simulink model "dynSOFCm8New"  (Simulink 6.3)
settings: Solver=ode15s  StartTime=0.0  StopTime=5000  FixedStep=0.001  MinStep=1e-12  RelTol=1e-3
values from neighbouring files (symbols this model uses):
  C = 300e-2    (= 3)    [dynSOFC_par.m]
  Cpc = 740    [dynSOFC_par.m]
  Cpt = 1217.7    [dynSOFC_par.m]
  D_a = 0.273*2*r3    (= 0.006006)    [dynSOFC_par.m]
  D_c = 2*(r2-r1)    (= 0.00532)    [dynSOFC_par.m]
  delta = 5.67e-8    (= 5.67e-08)    [dynSOFC_par.m]
  Ea = 1.1e5    (= 110000)    [dynSOFC_par.m]
  Ec = 1.2e5    (= 120000)    [dynSOFC_par.m]
  Ems1 = 0.4    [dynSOFC_par.m]
  Ems2 = 0.9    [dynSOFC_par.m]
  F = 96487    [dynSOFC_par.m]
  F21 = 0.69    [dynSOFC_par.m]
  K = 10    [dynSOFC_par.m]
  L = 1.5    [dynSOFC_par.m]
  La = 0.1e-3    (= 0.0001)    [dynSOFC_par.m]
  Lc = 2.21e-3    (= 0.00221)    [dynSOFC_par.m]
  Le = 0.04e-3    (= 4e-05)    [dynSOFC_par.m]
  R = 8.314/101325    (= 8.20528003948e-05)    [dynSOFC_par.m]
  r0 = 5e-3    (= 0.005)    [dynSOFC_par.m]
  r1 = 6e-3    (= 0.006)    [dynSOFC_par.m]
  r2 = 8.66e-3    (= 0.00866)    [dynSOFC_par.m]
  r3 = 11e-3    (= 0.011)    [dynSOFC_par.m]
  Ro = 1e-6    (= 1e-06)    [dynSOFC_par.m]
  Rouc = 4592    [dynSOFC_par.m]
  Rout = 3900    [dynSOFC_par.m]
  X = z(i)    [Simulate.m]    (also in dynSOFC_par.m = 0)
  x_ini = x_INI(i,:)    [Simulate.m]    (also in dynSOFC_par.m = [)
  XCH4 = 0.173    [dynSOFC_par.m]
  XCO = 0.057    [dynSOFC_par.m]
  XCO2 = 0.228    [dynSOFC_par.m]
  XH2 = 0.258    [dynSOFC_par.m]
  XH2O = 0.284    [dynSOFC_par.m]
  XO2 = 0.21    [dynSOFC_par.m]
libraries: simulink x23
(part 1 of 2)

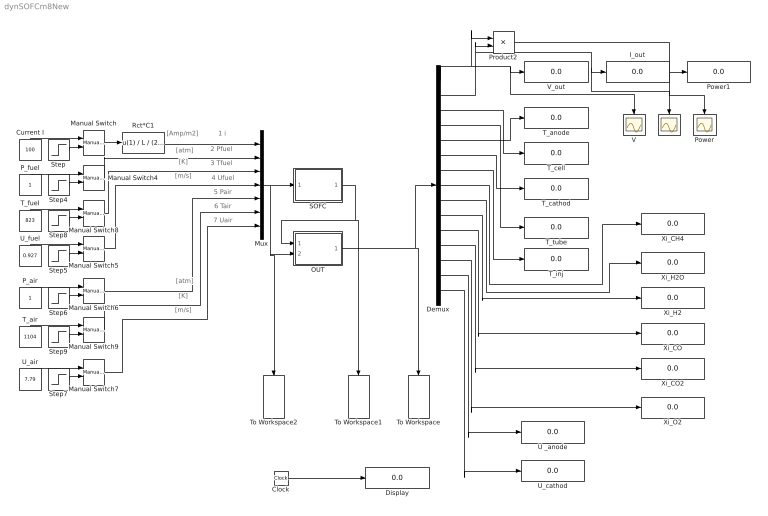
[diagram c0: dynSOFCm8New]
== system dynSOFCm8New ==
  note: [Amp/m2]
  note: [m/s]
  note: [atm]
  note: 1 i
  note: 3 Tfuel
  note: [K]
  note: 4 Ufuel
  note: 2 Pfuel
  note: 5 Pair
  note: 6 Tair
  note: 7 Uair
  note: [m/s]
  note: [K]
  note: [atm]
  Clock : Clock
  Current I : Constant  Orientation=up  Value=100
  Demux : Demux  Outputs=15
  Display : Display
  I : Scope
  I_out : Display
  Manual Switch{,4..6,8..9} (6 alike) : simulink/Signal Routing/Manual Switch  sw=1  action=0
  Manual Switch7 : simulink/Signal Routing/Manual Switch  sw=0  action=0
  Mux : Mux  Inputs=7
  OUT : Subsystem
  P_air : Constant  Orientation=up
  P_fuel : Constant  Orientation=up
  Power : Scope
  Power1 : Display
  Product2 : Product
  Rct*C1 : Fcn  Expr=u(1) / L / (2*pi*r3)
  SOFC : Subsystem
  Step : Step  Time=100  Before=100  After=200
  Step4 : Step  Time=100  Before=1  After=2
  Step5 : Step  Time=100  Before=0.97  After=2
  Step6 : Step  Time=100  Before=1  After=2
  Step7 : Step  Time=100  Before=7.79  After=23.37
  Step8 : Step  Time=100  Before=823  After=923
  Step9 : Step  Time=100  Before=1104  After=1204
  T_air : Constant  Orientation=up  Value=1104
  T_anode : Display
  T_cathod : Display
  T_cell : Display
  T_fuel : Constant  Orientation=up  Value=823
  T_inj : Display
  T_tube : Display
  To Workspace : ToWorkspace  VariableName=y  SampleTime=-1  SaveFormat=Array
  To Workspace1 : ToWorkspace  VariableName=x  SampleTime=-1  SaveFormat=Array
  To Workspace2 : ToWorkspace  VariableName=u  SaveFormat=Array
  U _anode : Display
  U_air : Constant  Orientation=up  Value=7.79
  U_cathod : Display
  U_fuel : Constant  Orientation=up  Value=0.927
  V : Scope
  V_out : Display
  Xi_CH4 : Display
  Xi_CO : Display
  Xi_CO2 : Display
  Xi_H2 : Display
  Xi_H2O : Display
  Xi_O2 : Display
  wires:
  Mux/1 -> SOFC/1(u), OUT/2(u), To Workspace2/1
  SOFC/1(x) -> OUT/1(x), To Workspace1/1
  OUT/1(y) -> Demux/1, To Workspace/1
  Demux/1 -> Product2/1, V_out/1, V/1
  Demux/2 -> Product2/2, I_out/1, I/1
  Current I/1 -> Manual Switch/1
  Step/1 -> Manual Switch/2
  Clock/1 -> Display/1
  P_fuel/1 -> Manual Switch4/1
  Step4/1 -> Manual Switch4/2
  U_fuel/1 -> Manual Switch5/1
  Step5/1 -> Manual Switch5/2
  P_air/1 -> Manual Switch6/1
  Step6/1 -> Manual Switch6/2
  U_air/1 -> Manual Switch7/1
  Step7/1 -> Manual Switch7/2
  T_fuel/1 -> Manual Switch8/1
  Step8/1 -> Manual Switch8/2
  T_air/1 -> Manual Switch9/1
  Step9/1 -> Manual Switch9/2
  Manual Switch5/1 -> Mux/4
  Manual Switch4/1 -> Mux/2
  Manual Switch8/1 -> Mux/3
  Manual Switch6/1 -> Mux/5
  Manual Switch9/1 -> Mux/6
  Manual Switch7/1 -> Mux/7
  Product2/1 -> Power1/1, Power/1
  Demux/3 -> T_cell/1
  Demux/4 -> T_tube/1
  Demux/5 -> T_anode/1
  Demux/6 -> T_cathod/1
  Demux/7 -> T_inj/1
  Demux/8 -> Xi_CH4/1
  Demux/9 -> Xi_H2O/1
  Demux/10 -> Xi_H2/1
  Demux/11 -> Xi_CO/1
  Demux/12 -> Xi_CO2/1
  Demux/13 -> Xi_O2/1
  Demux/14 -> U _anode/1
  Demux/15 -> U_cathod/1
  Manual Switch/1 -> Rct*C1/1
  Rct*C1/1 -> Mux/1

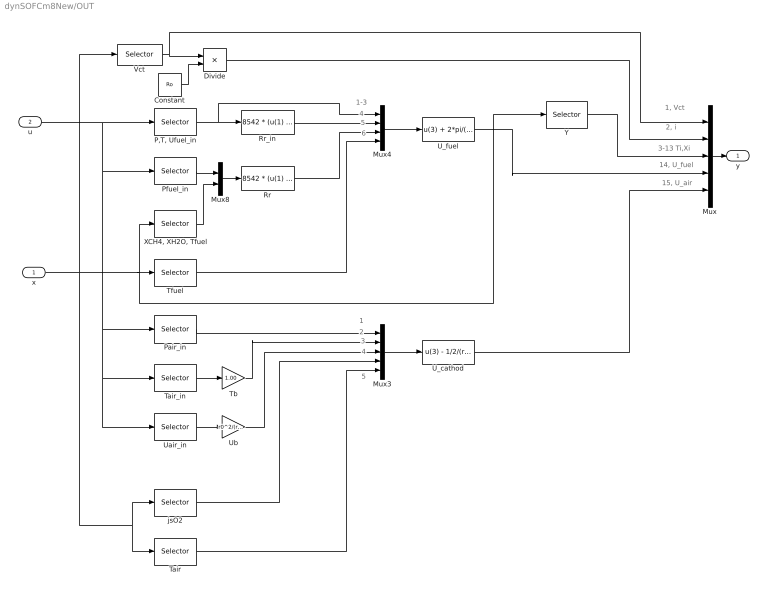
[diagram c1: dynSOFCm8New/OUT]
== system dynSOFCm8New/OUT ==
  note: 1-3
  note: 4
  note: 5
  note: 6
  note: 1
  note: 2
  note: 3
  note: 4
  note: 5
  note: 1, Vct
  note: 2, i
  note: 3-13 Ti,Xi
  note: 14, U_fuel
  note: 15, U_air
  x : Inport
  u : Inport  Port=2
  Constant : Constant  Value=Ro
  Divide : Product  Inputs=*/
  Mux : Mux  Inputs=5
  Mux3 : Mux  Inputs=5
  Mux4 : Mux
  Mux8 : Mux  Inputs=2
  "P,T, Ufuel_in" : Selector  Elements=[2 3 4]  InputPortWidth=7
  Pair_in : Selector  Elements=[5]  InputPortWidth=7
  Pfuel_in : Selector  Elements=[2]  InputPortWidth=7
  Rr : Fcn  Expr=8542 * (u(1) * u(2))^(0.85) * (u(1) * u(3))^(-0.35) * exp( -95e3 /(8.314*u(4)) )
  Rr_in : Fcn  Expr=8542 * (u(1) * XCH4)^(0.85) * (u(1) * XH2O)^(-0.35) * exp( -95e3 /(8.314*u(2)) )
  Tair : Selector  Elements=[18]  InputPortWidth=25
  Tair_in : Selector  Elements=[6]  InputPortWidth=7
  Tb : Gain  Gain=1.00
  Tfuel : Selector  Elements=[17]  InputPortWidth=25
  U_cathod : Fcn  Expr="u(3) - 1/2/(r2^2-r1^2)*(2*r1)  * R/u(1) * u(4) * ( u(2) + u(5)  ) * X"
  U_fuel : Fcn  Expr="u(3) + 2*pi/(4-pi)/r3  * R/u(1) * ( u(2) * u(4) + u(5) * u(6) ) * X"
  Uair_in : Selector  Elements=[7]  InputPortWidth=7
  Ub : Gain  Gain=r0^2/(r2^2-r1^2)
  Vct : Selector  Elements=[1]  InputPortWidth=25
  "XCH4, XH2O, Tfuel" : Selector  Elements=[20 21 17]  InputPortWidth=25
  Y : Selector  Elements=[15 16 17 18 19 20 21 22 23 24 25]  InputPortWidth=25
  jsO2 : Selector  Elements=[4]  InputPortWidth=25
  y : Outport
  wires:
  u/1 -> "P,T, Ufuel_in"/1, Pfuel_in/1, Pair_in/1, Uair_in/1, Tair_in/1
  Mux/1 -> y/1
  Tfuel/1 -> Mux4/4
  Pfuel_in/1 -> Mux8/1
  "XCH4, XH2O, Tfuel"/1 -> Mux8/2
  Mux8/1 -> Rr/1
  x/1 -> jsO2/1, Tair/1, Vct/1, "XCH4, XH2O, Tfuel"/1, Tfuel/1, Y/1
  "P,T, Ufuel_in"/1 -> Rr_in/1, Mux4/1
  Rr/1 -> Mux4/3
  Rr_in/1 -> Mux4/2
  Mux4/1 -> U_fuel/1
  Vct/1 -> Divide/1, Mux/1
  Constant/1 -> Divide/2
  jsO2/1 -> Mux3/4
  Pair_in/1 -> Mux3/1
  Mux3/1 -> U_cathod/1
  Uair_in/1 -> Ub/1
  Tair/1 -> Mux3/5
  Ub/1 -> Mux3/3
  Tair_in/1 -> Tb/1
  Tb/1 -> Mux3/2
  Divide/1 -> Mux/2
  Y/1 -> Mux/3
  U_fuel/1 -> Mux/4
  U_cathod/1 -> Mux/5

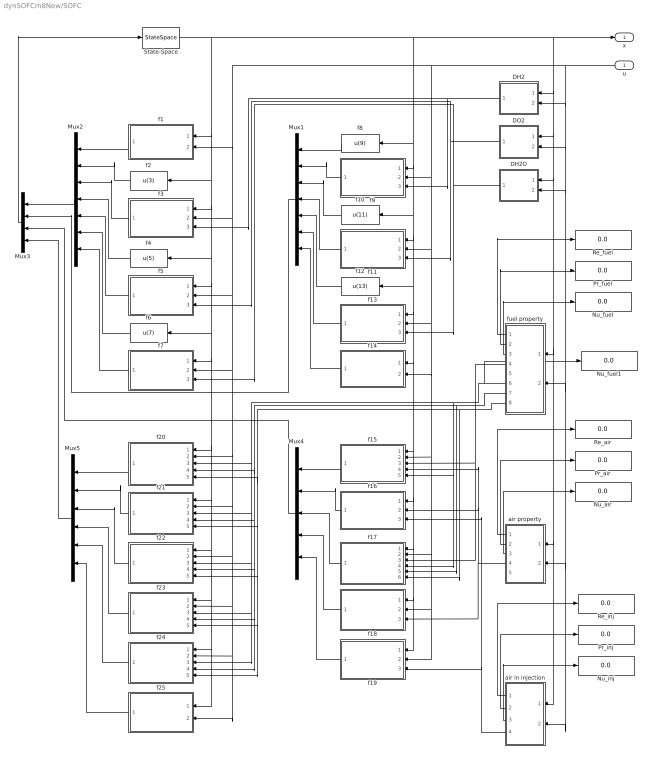
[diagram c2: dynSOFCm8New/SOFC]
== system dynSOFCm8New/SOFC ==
  u : Inport  Orientation=left
  DH2 : Subsystem  Orientation=left
  DH2O : Subsystem  Orientation=left
  DO2 : Subsystem  Orientation=left
  Mux1 : Mux  Orientation=left  Inputs=7
  Mux2 : Mux  Orientation=left  Inputs=7
  Mux3 : Mux  Orientation=left
  Mux4 : Mux  Orientation=left  Inputs=5
  Mux5 : Mux  Orientation=left  Inputs=6
  Nu_air : Display
  Nu_fuel : Display
  Nu_fuel1 : Display
  Nu_inj : Display
  Pr_air : Display
  Pr_fuel : Display
  Pr_inj : Display
  Re_air : Display
  Re_fuel : Display
  Re_inj : Display
  State-Space : StateSpace  A=zeros(25,25)  B=eye(25,25)  C=eye(25,25)  D=zeros(25,25)  X0=x_ini
  air in injection : Subsystem  Orientation=left
  air property : Subsystem  Orientation=left
  f1 : Subsystem  Orientation=left
  f10 : Fcn  Orientation=left  Expr=u(11)
  f11 : Subsystem  Orientation=left
  f12 : Fcn  Orientation=left  Expr=u(13)
  f13 : Subsystem  Orientation=left
  f14 : Subsystem  Orientation=left
  f15 : Subsystem  Orientation=left
  f16 : Subsystem  Orientation=left
  f17 : Subsystem  Orientation=left
  f18 : Subsystem  Orientation=left
  f19 : Subsystem  Orientation=left
  f2 : Fcn  Orientation=left  Expr=u(3)
  f20 : Subsystem  Orientation=left
  f21 : Subsystem  Orientation=left
  f22 : Subsystem  Orientation=left
  f23 : Subsystem  Orientation=left
  f24 : Subsystem  Orientation=left
  f25 : Subsystem  Orientation=left
  f3 : Subsystem  Orientation=left
  f4 : Fcn  Orientation=left  Expr=u(5)
  f5 : Subsystem  Orientation=left
  f6 : Fcn  Orientation=left  Expr=u(7)
  f7 : Subsystem  Orientation=left
  f8 : Fcn  Orientation=left  Expr=u(9)
  f9 : Subsystem  Orientation=left
  fuel property : Subsystem  Orientation=left
  x : Outport
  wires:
  State-Space/1 -> f1/1(x), f2/1, f3/1(x), f4/1, f6/1, f7/1(x), f21/1(x), f22/1(x), f23/1(x), f24/1(x), f25/1(x), f20/1(x), f5/1(x), f8/1, f9/1(x), f10/1, f11/1(x), f13/1(x), f14/1(x), f15/1(x), f16/1(x), f17/1(x), f18/1(x), f19/1(x), f12/1, x/1, DH2/1(x), DO2/1(x), DH2O/1(x), fuel property/1(x), air property/1(x), air in injection/1(x)
  f3/1(dot x3) -> Mux2/3
  f2/1 -> Mux2/2
  f1/1(dot x1) -> Mux2/1
  f4/1 -> Mux2/4
  f5/1(dot x5) -> Mux2/5
  f6/1 -> Mux2/6
  f7/1(dot x7) -> Mux2/7
  f8/1 -> Mux1/1
  f9/1(dot x9) -> Mux1/2
  f10/1 -> Mux1/3
  f11/1(dot x11) -> Mux1/4
  f12/1 -> Mux1/5
  f13/1(dot x13) -> Mux1/6
  f14/1(dot x14) -> Mux1/7
  Mux2/1 -> Mux3/1
  Mux3/1 -> State-Space/1
  u/1 -> f1/2(u), f3/2(u), f7/2(u), f21/2(u), f22/2(u), f23/2(u), f24/2(u), f25/2(u), f20/2(u), f5/2(u), f9/2(u), f13/2(u), f14/2(u), f15/2(u), f17/2(u), f18/2(u), f19/2(u), f11/2(u), DH2/2(u), DO2/2(u), DH2O/2(u), fuel property/2(u), air property/2(u), air in injection/2(u)
  DH2/1(DH2) -> f3/3(DH2), f9/3(DH2)
  DO2/1(DO2) -> f11/3(DO2), f5/3(DO2)
  DH2O/1(DH2O) -> f7/3(DH2O), f13/3(DH2O)
  Mux1/1 -> Mux3/2
  fuel property/4(h_fuel) -> f15/3(ha), f17/3(ha)
  air in injection/4(h_inj) -> f19/3(ht), f16/3(h_t)
  f15/1(dot x15) -> Mux4/1
  f16/1(dot x16) -> Mux4/2
  f17/1(dot x17) -> Mux4/3
  f18/1(dot x18) -> Mux4/4
  f19/1(dot x19) -> Mux4/5
  f20/1(dot x20) -> Mux5/1
  f21/1(dot x21) -> Mux5/2
  f22/1(dot x22) -> Mux5/3
  f23/1(dot x23) -> Mux5/4
  f24/1(dot x24) -> Mux5/5
  Mux4/1 -> Mux3/3
  Mux5/1 -> Mux3/4
  air property/1(Re_air) -> Re_air/1
  air property/2(Pr_air) -> Pr_air/1
  fuel property/1(Re_fuel) -> Re_fuel/1
  fuel property/2(Pr_fuel) -> Pr_fuel/1
  fuel property/3(Nu_fuel) -> Nu_fuel/1
  air in injection/1(Re_inj) -> Re_inj/1
  air in injection/2(Pr_inj) -> Pr_inj/1
  f25/1(dot x25) -> Mux5/6
  air property/4(h_air) -> f18/3(hc), f16/2(hc), f15/4(hc)
  fuel property/6(r_ref) -> Nu_fuel1/1, f15/5(r_ref), f17/4(r_ref), f21/3(r_ref), f22/3(r_ref), f23/3(r_ref), f24/3(r_ref), f20/3(r_ref)
  fuel property/7(r_sft) -> f17/5(r_sft), f21/4(r_sft), f22/4(r_sft), f23/4(r_sft), f24/4(r_sft), f20/4(r_sft)
  fuel property/8(r_ref_in) -> f17/6(r_ref_in), f21/5(r_ref_in), f22/5(r_ref_in), f23/5(r_ref_in), f24/5(r_ref_in), f20/5(r_ref_in)
  air in injection/3(Nu_inj) -> Nu_inj/1
  air property/3(Nu_air) -> Nu_air/1

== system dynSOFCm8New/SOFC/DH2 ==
  x : Inport
  u : Inport  Port=2
  D : Fcn  Expr=4.17e-5*u(1)^1.75/u(2)/101325
  Mux1 : Mux  Inputs=2
  Pfuel : Selector  Elements=[2]  InputPortWidth=7
  Tcell : Selector  Elements=[15]  InputPortWidth=25
  DH2 : Outport
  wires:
  Pfuel/1 -> Mux1/2
  u/1 -> Pfuel/1
  x/1 -> Tcell/1
  Tcell/1 -> Mux1/1
  Mux1/1 -> D/1
  D/1 -> DH2/1

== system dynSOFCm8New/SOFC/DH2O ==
  x : Inport
  u : Inport  Port=2
  D : Fcn  Expr=4.17e-5*u(1)^1.75/u(2)/101325
  Mux1 : Mux  Inputs=2
  Pfuel : Selector  Elements=[2]  InputPortWidth=7
  Tcell : Selector  Elements=[15]  InputPortWidth=25
  DH2O : Outport
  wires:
  D/1 -> DH2O/1
  Mux1/1 -> D/1
  Tcell/1 -> Mux1/1
  x/1 -> Tcell/1
  u/1 -> Pfuel/1
  Pfuel/1 -> Mux1/2

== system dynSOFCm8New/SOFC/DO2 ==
  x : Inport
  u : Inport  Port=2
  D : Fcn  Expr=9.82e-6*u(1)^1.75/u(2)/101325
  Mux1 : Mux  Inputs=2
  Pair : Selector  Elements=[5]  InputPortWidth=7
  Tcell : Selector  Elements=[15]  InputPortWidth=25
  DO2 : Outport
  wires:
  D/1 -> DO2/1
  Mux1/1 -> D/1
  Tcell/1 -> Mux1/1
  x/1 -> Tcell/1
  u/1 -> Pair/1
  Pair/1 -> Mux1/2

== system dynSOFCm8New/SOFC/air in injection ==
  note: u7
  note: u5
  note: x19
  x : Inport
  u : Inport  Port=2
  Density : Fcn  Expr=u(3) * u(2)/(R*u(1)) / 1000
  Mux2 : Mux  Inputs=3
  Mux3 : Mux  Inputs=3
  Mux4 : Mux
  Mux5 : Mux  Orientation=left  Inputs=2
  Mux6 : Mux  Inputs=2
  Nusselt number : Fcn  Expr=0.332*u(2)^(1/3)*u(1)^(1/2)
  P_inj : Selector  Elements=[5]  InputPortWidth=7
  Prandtl number : Fcn  Expr=u(3)/u(1)*u(2)/u(4)
  Renold number : Fcn  Expr=D_c*u(1)*u(2)/u(3)
  T_air : Selector  Elements=[19]  InputPortWidth=25
  U_air : Selector  Elements=[7]  InputPortWidth=7
  conductivity : Fcn  Expr=0.01329 + 5.539e-5*u(1)
  "heat capacity, Cp" : Fcn  Expr=2.779e4 + 4.936*u(1)
  heat transfer coefficient : Fcn  Expr=u(1)*u(2)/D_c
  mole mass : Constant  Value=29
  viscosity : Fcn  Expr=1.514e-5 + 2.793e-8*u(1)
  Re_inj : Outport
  Pr_inj : Outport  Port=2
  Nu_inj : Outport  Port=3
  h_inj : Outport  Port=4
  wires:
  u/1 -> P_inj/1, U_air/1
  Nusselt number/1 -> Nu_inj/1, Mux6/1
  Mux5/1 -> Nusselt number/1
  Prandtl number/1 -> Mux5/2, Pr_inj/1
  conductivity/1 -> Mux4/4, Mux6/2
  "heat capacity, Cp"/1 -> Mux4/3
  Mux4/1 -> Prandtl number/1
  viscosity/1 -> Mux4/2, Mux3/3
  mole mass/1 -> Mux4/1, Mux2/3
  P_inj/1 -> Mux2/2
  Renold number/1 -> Mux5/1, Re_inj/1
  Mux3/1 -> Renold number/1
  Density/1 -> Mux3/2
  Mux2/1 -> Density/1
  U_air/1 -> Mux3/1
  T_air/1 -> Mux2/1, "heat capacity, Cp"/1, conductivity/1, viscosity/1
  Mux6/1 -> heat transfer coefficient/1
  heat transfer coefficient/1 -> h_inj/1
  x/1 -> T_air/1

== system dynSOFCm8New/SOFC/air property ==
  note: u7
  note: x25,18
  note: u5
  x : Inport
  u : Inport  Port=2
  Density : Fcn  Expr="((1-u(1)) *28 + u(1)*32) * u(3)/(R*u(2))  /1000"
  Mole Mass : Fcn  Expr=(1 - u(1)) *28 + u(1)*32
  Mux1 : Mux  Inputs=2
  Mux3 : Mux  Inputs=3
  Mux4 : Mux
  Mux5 : Mux  Orientation=left  Inputs=2
  Mux6 : Mux  Inputs=2
  Nusselt number : Fcn  Expr=0.332*u(2)^(1/3)*u(1)^(1/2)
  P_air_in : Selector  Elements=[5]  InputPortWidth=7
  Prandtl number : Fcn  Expr=u(3)/u(1)*u(2)/u(4)
  Renold number : Fcn  Expr=D_c*u(1)*u(2)/u(3)
  U_air_in : Selector  Elements=[7]  InputPortWidth=7
  Ub : Gain  Gain=r0^2/(r2^2-r1^2)
  XO2,T_air : Selector  Elements=[25,18]  InputPortWidth=25
  conductivity : Fcn  Expr=0.01329 + 5.539e-5*u(2)
  "heat capacity, Cp" : Fcn  Expr=2.779e4 + 4.936*u(2)
  heat transfer coefficient : Fcn  Expr=u(1)*u(2)/D_c
  viscosity : Fcn  Expr=1.514e-5 + 2.793e-8*u(2)
  Re_air : Outport
  Pr_air : Outport  Port=2
  Nu_air : Outport  Port=3
  h_air : Outport  Port=4
  "Cp, air" : Outport  Port=5
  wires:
  heat transfer coefficient/1 -> h_air/1
  Mux6/1 -> heat transfer coefficient/1
  Density/1 -> Mux3/2
  Mux3/1 -> Renold number/1
  Renold number/1 -> Re_air/1, Mux5/1
  x/1 -> XO2,T_air/1
  Mole Mass/1 -> Mux4/1
  viscosity/1 -> Mux3/3, Mux4/2
  Mux4/1 -> Prandtl number/1
  "heat capacity, Cp"/1 -> Mux4/3, "Cp, air"/1
  conductivity/1 -> Mux6/2, Mux4/4
  Prandtl number/1 -> Pr_air/1, Mux5/2
  Mux5/1 -> Nusselt number/1
  Nusselt number/1 -> Mux6/1, Nu_air/1
  Mux1/1 -> Mole Mass/1, viscosity/1, "heat capacity, Cp"/1, conductivity/1, Density/1
  XO2,T_air/1 -> Mux1/1
  u/1 -> U_air_in/1, P_air_in/1
  P_air_in/1 -> Mux1/2
  U_air_in/1 -> Ub/1
  Ub/1 -> Mux3/1

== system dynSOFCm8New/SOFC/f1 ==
  note: E-Vct
  note: Tcell
  note: Vct
  note: i
  x : Inport
  u : Inport  Port=2
  Divide : Product  Inputs=*/
  E : Subsystem
  Gain1 : Gain  Gain=1/C
  I : Selector  Elements=[1]  InputPortWidth=7
  Rct*C : Fcn  Expr=2.94e-5*exp(10350/u(1)) *Le*C
  Sum : Sum  Inputs=|+-
  Sum1 : Sum  Inputs=|+-
  Tcell : Selector  Elements=[15]  InputPortWidth=25
  Vct : Selector  Elements=[1]  InputPortWidth=25
  dot x1 : Outport
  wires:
  E/1(E) -> Sum/1
  x/1 -> Vct/1, Tcell/1, E/1(x)
  Vct/1 -> Sum/2
  u/1 -> I/1, E/2(u)
  Gain1/1 -> Sum1/2
  Sum1/1 -> dot x1/1
  Sum/1 -> Divide/1
  Divide/1 -> Sum1/1
  Tcell/1 -> Rct*C/1
  Rct*C/1 -> Divide/2
  I/1 -> Gain1/1

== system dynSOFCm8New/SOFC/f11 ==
  note: 1-4
  note: 5
  note: 6
  note: 7-10
  note: x10,11,14,15
  note: u1
  note: x25
  note: u5
  note: pbO2
  note: dot ptO2
  note: ptO2
  note: i
  note: Vi
  note: Tcell
  x : Inport
  u : Inport  Port=2
  DO2 : Inport  Port=3
  Ex11 : Fcn  Expr="-u(7)*u(1) - u(8)*u(2)  + u(7)*u(5) - R*u(4)/(4*F)*( u(10)*u(6) + 4/Lc*(K*u(6)-u(3)) )"
  Mux : Mux
  Mux3 : Mux
  Mux4 : Mux  Inputs=2
  Pair_in : Selector  Elements=[5]  InputPortWidth=7
  XO2 : Selector  Elements=[25 ]  InputPortWidth=25
  a1 : Fcn  Expr=24*u(1)^2/(Lc^4)
  a2 : Fcn  Expr=12*u(1)/(Lc^2)
  a3 : Fcn  Expr=24*u(1)^2/(Lc^3)
  a4 : Fcn  Expr=24*u(1)/(Lc^3)
  i : Selector  Elements=[1]  InputPortWidth=7
  pbO2 : Fcn  Expr=u(2)*u(1)
  ptO2 : Selector  Elements=[10 11 14 15]  InputPortWidth=25
  dot x11 : Outport
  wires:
  DO2/1 -> a1/1, a2/1, a4/1, a3/1
  a1/1 -> Mux/1
  a2/1 -> Mux/2
  a3/1 -> Mux/3
  a4/1 -> Mux/4
  x/1 -> ptO2/1, XO2/1
  Mux3/1 -> Ex11/1
  Ex11/1 -> dot x11/1
  pbO2/1 -> Mux3/2
  u/1 -> Pair_in/1, i/1
  ptO2/1 -> Mux3/1
  XO2/1 -> Mux4/1
  Pair_in/1 -> Mux4/2
  Mux4/1 -> pbO2/1
  i/1 -> Mux3/3
  Mux/1 -> Mux3/4

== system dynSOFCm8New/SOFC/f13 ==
  note: 1-4
  note: 5
  note: 6
  note: 7-10
  note: x12,13,14,15
  note: u1
  note: x21
  note: u2
  note: pbH2O
  note: dot ptH2O
  note: ptH2O
  note: i
  note: Vi
  note: Tcell
  x : Inport
  u : Inport  Port=2
  DH2O : Inport  Port=3
  Ex9 : Fcn  Expr="-u(7)*u(1) - u(8)*u(2)  + u(7)*u(5) - R*u(4)/(2*F)*( u(10)*(-u(6)) - 4/La*(K*u(6)-u(3)) )"
  Mux : Mux
  Mux2 : Mux
  Mux4 : Mux  Inputs=2
  Pfuel_in : Selector  Elements=[2]  InputPortWidth=7
  XH2O : Selector  Elements=[21 ]  InputPortWidth=25
  a1 : Fcn  Expr=24*u(1)^2/(La^4)
  a2 : Fcn  Expr=12*u(1)/(La^2)
  a3 : Fcn  Expr=24*u(1)^2/(La^3)
  a4 : Fcn  Expr=24*u(1)/(La^3)
  i : Selector  Elements=[1]  InputPortWidth=7
  pbH2O : Fcn  Expr=u(2)*u(1)
  ptH2 : Selector  Elements=[12 13 14 15]  InputPortWidth=25
  dot x13 : Outport
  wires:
  DH2O/1 -> a1/1, a2/1, a4/1, a3/1
  a1/1 -> Mux/1
  a2/1 -> Mux/2
  a3/1 -> Mux/3
  a4/1 -> Mux/4
  x/1 -> ptH2/1, XH2O/1
  Mux2/1 -> Ex9/1
  Ex9/1 -> dot x13/1
  pbH2O/1 -> Mux2/2
  u/1 -> Pfuel_in/1, i/1
  ptH2/1 -> Mux2/1
  XH2O/1 -> Mux4/1
  Pfuel_in/1 -> Mux4/2
  Mux4/1 -> pbH2O/1
  i/1 -> Mux2/3
  Mux/1 -> Mux2/4

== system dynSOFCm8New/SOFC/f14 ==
  x : Inport
  u : Inport  Port=2
  Gain : Gain  Gain=K
  Gain1 : Gain  Gain=K^2
  Selector : Selector  Elements=[14]  InputPortWidth=25
  Selector1 : Selector  Elements=[1]  InputPortWidth=7
  Sum : Sum  Inputs=|-+
  dot x14 : Outport
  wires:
  Gain1/1 -> Sum/2
  Gain/1 -> Sum/1
  Selector1/1 -> Gain1/1
  Selector/1 -> Gain/1
  u/1 -> Selector1/1
  x/1 -> Selector/1
  Sum/1 -> dot x14/1

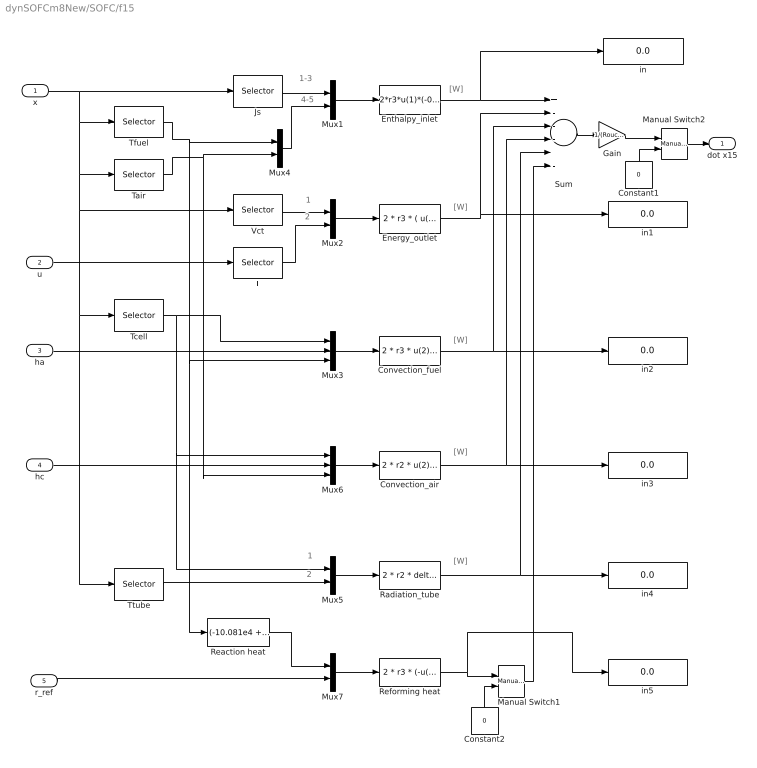
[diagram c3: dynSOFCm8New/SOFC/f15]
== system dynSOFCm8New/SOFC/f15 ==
  note: 1-3
  note: 4-5
  note: 1
  note: 2
  note: 1
  note: 2
  note: [W]
  note: [W]
  note: [W]
  note: [W]
  note: [W]
  x : Inport
  u : Inport  Port=2
  ha : Inport  Port=3
  hc : Inport  Port=4
  r_ref : Inport  Port=5
  Constant1 : Constant  Orientation=up  Value=0
  Constant2 : Constant  Orientation=up  Value=0
  Convection_air : Fcn  Expr=2 * r2 * u(2) * (u(1) - u(3))
  Convection_fuel : Fcn  Expr=2 * r3 * u(2) * (u(1) - u(3))
  Energy_outlet : Fcn  Expr=2 * r3 * ( u(1)*u(2) - u(2)^2 * Ro )
  Enthalpy_inlet : Fcn  Expr="2*r3*u(1)*(-0.9959e4+30.73*u(4)) + 2*r2*u(2)*(-1.2290e4+35.12*u(5))  + 2*r3*u(3)*(-25.790e4+42.47*u(4))"
  Gain : Gain  Gain=1/(Rouc*Cpc*(r3^2-r2^2))
  I : Selector  Elements=[1]  InputPortWidth=7
  Js : Selector  Elements=[2 4 6]  InputPortWidth=25
  Manual Switch1 : simulink/Signal Routing/Manual Switch  sw=1  action=0
  Manual Switch2 : simulink/Signal Routing/Manual Switch  sw=1  action=0
  Mux{1..2,4..5,7} (5 alike) : Mux  Inputs=2
  Mux3 : Mux  Inputs=3
  Mux6 : Mux  Inputs=3
  Radiation_tube : Fcn  Expr=2 * r2 * delta*(u(1)^4-u(2)^4)/((1-Ems2)/Ems2 + 1/F21 + (1-Ems1)/Ems1*(r2/r1)^2)
  Reaction heat : Fcn  Expr="(-10.081e4 + 62.12 * u(1)) +  (-25.79e4 + 42.47 * u(1)) - 3* (-0.9959e4 + 30.73*u(1))  -  (-12.150e4 + 31.81* u(1))"
  Reforming heat : Fcn  Expr=2 * r3 * (-u(1) * u(2))
  Sum : Sum  Inputs=+-----
  Tair : Selector  Elements=[18]  InputPortWidth=25
  Tcell : Selector  Elements=[15]  InputPortWidth=25
  Tfuel : Selector  Elements=[17]  InputPortWidth=25
  Ttube : Selector  Elements=[16]  InputPortWidth=25
  Vct : Selector  Elements=[1]  InputPortWidth=25
  in{,1..5} (6 alike) : Display
  dot x15 : Outport
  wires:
  x/1 -> Js/1, Tfuel/1, Vct/1, Tcell/1, Ttube/1, Tair/1
  Js/1 -> Mux1/1
  Mux1/1 -> Enthalpy_inlet/1
  Mux4/1 -> Mux1/2
  Vct/1 -> Mux2/1
  I/1 -> Mux2/2
  Mux2/1 -> Energy_outlet/1
  Mux3/1 -> Convection_fuel/1
  Mux5/1 -> Radiation_tube/1
  Tcell/1 -> Mux3/1, Mux5/1, Mux6/1
  u/1 -> I/1
  Enthalpy_inlet/1 -> Sum/1, in/1
  Energy_outlet/1 -> Sum/2, in1/1
  Convection_fuel/1 -> Sum/3, in2/1
  Convection_air/1 -> Sum/4, in3/1
  Radiation_tube/1 -> Sum/5, in4/1
  Mux6/1 -> Convection_air/1
  Tfuel/1 -> Mux4/1, Mux3/3, Reaction heat/1
  ha/1 -> Mux3/2
  hc/1 -> Mux6/2
  Tair/1 -> Mux6/3, Mux4/2
  Ttube/1 -> Mux5/2
  Mux7/1 -> Reforming heat/1
  r_ref/1 -> Mux7/2
  Reaction heat/1 -> Mux7/1
  Sum/1 -> Gain/1
  Gain/1 -> Manual Switch2/1
  Constant1/1 -> Manual Switch2/2
  Manual Switch2/1 -> dot x15/1
  Reforming heat/1 -> Manual Switch1/1, in5/1
  Constant2/1 -> Manual Switch1/2
  Manual Switch1/1 -> Sum/6

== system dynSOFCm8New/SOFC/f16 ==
  note: [W]
  note: [W]
  note: [W]
  x : Inport
  hc : Inport  Port=2
  h_t : Inport  Port=3
  Constant1 : Constant  Orientation=up  Value=0
  Convection_air : Fcn  Expr=2 * r1 * u(3) * (u(2) - u(1))
  Convection_inj : Fcn  Expr="2 * r0 *  u(3) * (u(1) - u(2))"
  Gain : Gain  Gain=1/(Rout*Cpt*(r1^2-r0^2))
  Manual Switch2 : simulink/Signal Routing/Manual Switch  sw=1  action=0
  Mux3 : Mux  Inputs=3
  Mux5 : Mux  Inputs=2
  Mux6 : Mux  Inputs=3
  Radiation_tube : Fcn  Expr=2 *r2 * delta*(u(1)^4-u(2)^4)/((1-Ems2)/Ems2 + 1/F21 + (1-Ems1)/Ems1*(r2/r1)^2)
  Sum : Sum  Inputs=+--
  Tair : Selector  Elements=[18]  InputPortWidth=25
  Tcell : Selector  Elements=[15]  InputPortWidth=25
  Tinj : Selector  Elements=[19]  InputPortWidth=25
  Ttube : Selector  Elements=[16]  InputPortWidth=25
  in1 : Display
  in2 : Display
  in3 : Display
  dot x16 : Outport
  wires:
  Mux6/1 -> Convection_inj/1
  Radiation_tube/1 -> in1/1, Sum/1
  Convection_inj/1 -> in3/1, Sum/3
  Convection_air/1 -> in2/1, Sum/2
  Mux5/1 -> Radiation_tube/1
  Mux3/1 -> Convection_air/1
  x/1 -> Tcell/1, Tair/1, Tinj/1, Ttube/1
  Tair/1 -> Mux3/1
  Tcell/1 -> Mux5/1
  Ttube/1 -> Mux5/2, Mux3/2, Mux6/1
  hc/1 -> Mux3/3
  Tinj/1 -> Mux6/2
  h_t/1 -> Mux6/3
  Sum/1 -> Gain/1
  Constant1/1 -> Manual Switch2/2
  Gain/1 -> Manual Switch2/1
  Manual Switch2/1 -> dot x16/1

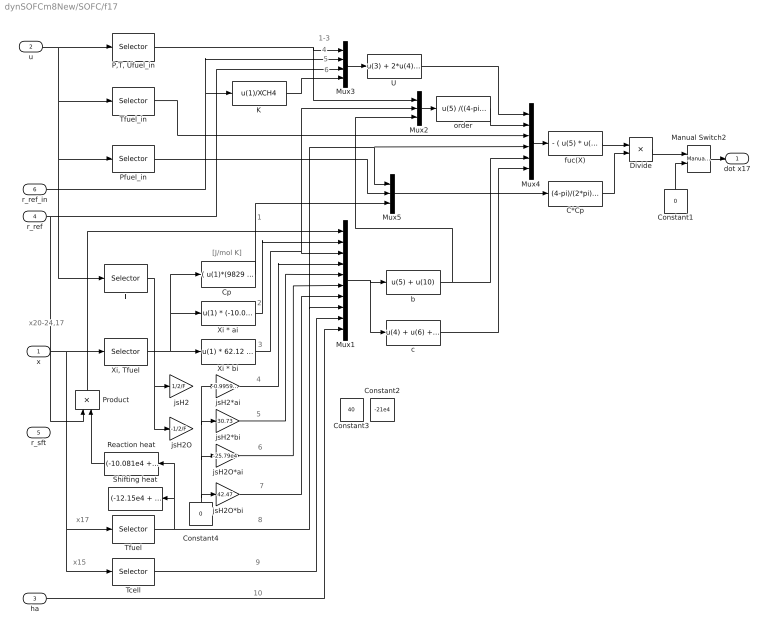
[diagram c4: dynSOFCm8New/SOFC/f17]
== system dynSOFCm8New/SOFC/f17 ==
  note: x20-24,17
  note: x17
  note: x15
  note: 1
  note: 2
  note: 3
  note: 4
  note: 5
  note: 6
  note: 7
  note: 8
  note: 9
  note: 10
  note: 1-3
  note: 4
  note: 5
  note: 6
  note: [J/mol K]
  x : Inport
  u : Inport  Port=2
  ha : Inport  Port=3
  r_ref : Inport  Port=4
  r_sft : Inport  Port=5
  r_ref_in : Inport  Port=6
  C*Cp : Fcn  Expr="(4-pi)/(2*pi)*r3 * u(2) / ( R * u(1) )  * u(3)"
  Constant1 : Constant  Orientation=up  Value=0
  Constant2 : Constant  Orientation=up  Value=-21e4
  Constant3 : Constant  Orientation=up  Value=40
  Constant4 : Constant  Orientation=up  Value=0
  "Cp " : Fcn  Expr="( u(1)*(9829 + 83.47*u(6) -0.02053*u(6)^2)  + u(2)*(2.906e4 + 12.15*u(6)) +  u(3)*(2.660e4 +3.719*u(6)) + u(4)*(2.797e4 + 5.019*u(6)) + u(5)*(3.200e4 + 31.01*u(6) - 0.008875*u(6)^2) )  / 1000"
  Divide : Product  Inputs=*/
  K : Fcn  Expr=u(1)/XCH4
  Manual Switch2 : simulink/Signal Routing/Manual Switch  sw=1  action=0
  Mux1 : Mux  Inputs=10
  Mux2 : Mux  Inputs=3
  Mux3 : Mux
  Mux4 : Mux  Inputs=6
  Mux5 : Mux  Inputs=3
  "P,T, Ufuel_in" : Selector  Elements=[2 3 4]  InputPortWidth=7
  Pfuel_in : Selector  Elements=[2]  InputPortWidth=7
  Product : Product  Orientation=up
  Reaction heat : Fcn  Orientation=left  Expr="(-10.081e4 + 62.12 * u(1)) +  (-25.79e4 + 42.47 * u(1)) - 3* (-0.9959e4 + 30.73*u(1))  -  (-12.150e4 + 31.81* u(1))"
  Shifting heat : Fcn  Orientation=left  Expr="(-12.15e4 + 31.81 * u(1)) +  (-25.79e4 + 42.47 * u(1)) - (-0.9959e4 + 30.73*u(1))  -  (-41.700e4 + 50.89* u(1))"
  Tcell : Selector  Elements=[15]  InputPortWidth=25
  Tfuel : Selector  Elements=[17]  InputPortWidth=25
  Tfuel_in : Selector  Elements=[3]  InputPortWidth=7
  U : Fcn  Expr=u(3) + 2*u(4)*u(3)/u(6) * ( 1- exp( -X/((4-pi)/(2*pi)*r3 * u(1) /R/u(2) * u(3) / u(6)) ) )
  Xi * ai : Fcn  Expr="u(1) * (-10.081e4)  + u(2) * (-25.79e4 ) + u(3) * (-0.9959e4) + u(4) * (-12.150e4) + u(5) * (-41.700e4 )"
  Xi * bi : Fcn  Expr="u(1) * 62.12 + u(2) * 42.47  + u(3) * 30.73 + u(4) * 31.81 + u(5) * 50.89"
  "Xi, Tfuel" : Selector  Elements=[20 21 22 23 24 17]  InputPortWidth=25
  b : Fcn  Expr=u(5) + u(10)
  c : Fcn  Expr=u(4) + u(6) + ( u(7) - u(10) ) * u(9) - u(1)*0
  fuc(X) : Fcn  Expr=- ( u(5) * u(4) +u(6) ) + ( u(5) * u(3) +u(6) ) * exp( - u(2)*X/u(1) )
  i : Selector  Elements=[1]  InputPortWidth=7
  jsH2 : Gain  Gain=1/2/F
  jsH2*ai : Gain  Gain=-0.9959e4
  jsH2*bi : Gain  Gain=30.73
  jsH2O : Gain  Gain=-1/2/F
  jsH2O*ai : Gain  Gain=-25.79e4
  jsH2O*bi : Gain  Gain=42.47
  order : Fcn  Expr=u(5) /((4-pi)/(2*pi)*r3 * u(1) /R/u(2) * u(4))
  dot x17 : Outport
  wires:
  Tcell/1 -> Mux1/9
  "Xi, Tfuel"/1 -> Xi * bi/1, "Cp "/1, Xi * ai/1
  Tfuel/1 -> Mux1/8, Mux4/4, Mux5/1, Shifting heat/1, Reaction heat/1
  ha/1 -> Mux1/10
  Pfuel_in/1 -> Mux5/2
  jsH2O*bi/1 -> Mux1/7
  x/1 -> "Xi, Tfuel"/1, Tfuel/1, Tcell/1
  "P,T, Ufuel_in"/1 -> Mux3/1, Mux2/1
  u/1 -> "P,T, Ufuel_in"/1, Tfuel_in/1, Pfuel_in/1, i/1
  jsH2*ai/1 -> Mux1/4
  jsH2*bi/1 -> Mux1/5
  jsH2O*ai/1 -> Mux1/6
  Mux1/1 -> b/1, c/1
  Mux3/1 -> U/1
  Mux2/1 -> order/1
  b/1 -> Mux4/5, Mux2/3
  Mux4/1 -> fuc(X)/1
  U/1 -> Mux4/1
  order/1 -> Mux4/2
  Tfuel_in/1 -> Mux4/3
  c/1 -> Mux4/6
  Mux5/1 -> C*Cp/1
  fuc(X)/1 -> Divide/1
  C*Cp/1 -> Divide/2
  "Cp "/1 -> Mux5/3
  Divide/1 -> Manual Switch2/1
  Constant1/1 -> Manual Switch2/2
  Manual Switch2/1 -> dot x17/1
  i/1 -> jsH2/1, jsH2O/1
  r_ref/1 -> Mux3/3, Product/1
  r_ref_in/1 -> Mux3/2, K/1
  Product/1 -> Mux1/1
  K/1 -> Mux3/4
  Reaction heat/1 -> Product/2
  Constant4/1 -> jsH2O*bi/1, jsH2O*ai/1, jsH2*bi/1, jsH2*ai/1
  Xi * ai/1 -> Mux1/2
  Xi * bi/1 -> Mux1/3, Mux2/2

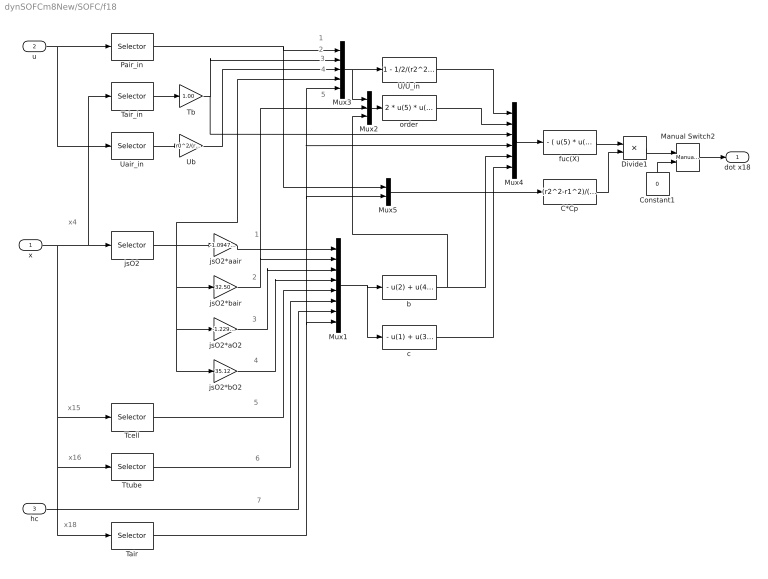
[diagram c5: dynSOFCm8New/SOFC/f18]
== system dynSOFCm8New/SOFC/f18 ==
  note: x4
  note: x15
  note: x16
  note: 1
  note: 4
  note: 5
  note: 6
  note: 7
  note: 1
  note: 2
  note: 3
  note: 4
  note: 2
  note: 3
  note: x18
  note: 5
  x : Inport
  u : Inport  Port=2
  hc : Inport  Port=3
  C*Cp : Fcn  Expr="(r2^2-r1^2)/(2*r1) * u(1) / ( R * u(2) )  * ( 2.7794e4 + 4.936 * u(2)) / 1000"
  Constant1 : Constant  Orientation=up  Value=0
  Divide1 : Product  Inputs=*/
  Manual Switch2 : simulink/Signal Routing/Manual Switch  sw=1  action=0
  Mux1 : Mux  Inputs=8
  Mux2 : Mux  Inputs=3
  Mux3 : Mux  Inputs=5
  Mux4 : Mux  Inputs=6
  Mux5 : Mux  Inputs=2
  Pair_in : Selector  Elements=[5]  InputPortWidth=7
  Tair : Selector  Elements=[18]  InputPortWidth=25
  Tair_in : Selector  Elements=[16]  InputPortWidth=25
  Tb : Gain  Gain=1.00
  Tcell : Selector  Elements=[15]  InputPortWidth=25
  Ttube : Selector  Elements=[16]  InputPortWidth=25
  U/U_in : Fcn  Expr="1 - 1/2/(r2^2-r1^2)*(2*r1)  * R/u(1)/u(3) * u(4) * ( u(2) + u(5)  ) * X"
  Uair_in : Selector  Elements=[7]  InputPortWidth=7
  Ub : Gain  Gain=r0^2/(r2^2-r1^2)
  b : Fcn  Expr=- u(2) + u(4) + u(7) + r2/r1*u(7)
  c : Fcn  Expr=- u(1) + u(3) - u(7)*u(5) - r2/r1*u(7)*u(6)
  fuc(X) : Fcn  Expr=- ( u(5) * u(4) +u(6) ) + ( u(5) * u(3) +u(6) ) * ( u(1) ^ u(2))
  jsO2 : Selector  Elements=[4]  InputPortWidth=25
  jsO2*aO2 : Gain  Gain=-1.229e4
  jsO2*aair : Gain  Gain=-1.0947e4
  jsO2*bO2 : Gain  Gain=35.12
  jsO2*bair : Gain  Gain=32.50
  order : Fcn  Expr="2 * u(5) * u(7) / ( u(6) * ( u(2)  + u(5) ) )"
  dot x18 : Outport
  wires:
  Ttube/1 -> Mux1/6
  Tcell/1 -> Mux1/5
  hc/1 -> Mux1/7
  jsO2/1 -> jsO2*aair/1, jsO2*bair/1, jsO2*aO2/1, jsO2*bO2/1, Mux3/4
  jsO2*bO2/1 -> Mux1/4
  x/1 -> Tcell/1, Ttube/1, Tair/1, jsO2/1, Tair_in/1
  Pair_in/1 -> Mux3/1, Mux5/1
  u/1 -> Pair_in/1, Uair_in/1
  jsO2*aair/1 -> Mux1/1
  jsO2*bair/1 -> Mux1/2, Mux2/2
  jsO2*aO2/1 -> Mux1/3
  Mux1/1 -> b/1, c/1
  Mux3/1 -> U/U_in/1, Mux2/1
  Mux2/1 -> order/1
  b/1 -> Mux2/3, Mux4/5
  Mux4/1 -> fuc(X)/1
  U/U_in/1 -> Mux4/1
  order/1 -> Mux4/2
  c/1 -> Mux4/6
  Mux5/1 -> C*Cp/1
  fuc(X)/1 -> Divide1/1
  C*Cp/1 -> Divide1/2
  Uair_in/1 -> Ub/1
  Tair/1 -> Mux1/8, Mux3/5, Mux4/4, Mux5/2
  Ub/1 -> Mux3/3
  Tair_in/1 -> Tb/1
  Tb/1 -> Mux3/2, Mux4/3
  Divide1/1 -> Manual Switch2/1
  Constant1/1 -> Manual Switch2/2
  Manual Switch2/1 -> dot x18/1

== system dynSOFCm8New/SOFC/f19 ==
  note: x19
  note: x16
  note: u5
  note: u6
  note: u7
  x : Inport
  u : Inport  Port=2
  ht : Inport  Port=3
  C*Cp : Fcn  Expr=r0/2 * u(1) / R / u(2) * ( 2.7794e4 + 4.936 * u(4)) / 1000
  Constant1 : Constant  Orientation=up  Value=0
  Divide : Product  Inputs=*/
  Manual Switch2 : simulink/Signal Routing/Manual Switch  sw=1  action=0
  Mux1 : Mux  Inputs=5
  Mux2 : Mux  Inputs=5
  Pair_in : Selector  Elements=[5]  InputPortWidth=7
  Tair_in : Selector  Elements=[6]  InputPortWidth=7
  Tinj : Selector  Elements=[19]  InputPortWidth=25
  Ttube : Selector  Elements=[16]  InputPortWidth=25
  Uair_in : Selector  Elements=[7]  InputPortWidth=7
  func : Fcn  Expr=u(4) * ( -u(2) + u(3) ) + u(4) * ( u(1) -u(3) ) * exp (u(5))
  in1 : Display
  order : Fcn  Expr=- 2/r0 * u(5) * R * u(4) / ( 32.5 * u(1) * u(3)) * (L-X)
  dot x19 : Outport
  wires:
  func/1 -> Divide/1
  u/1 -> Pair_in/1, Uair_in/1, Tair_in/1
  x/1 -> Tinj/1, Ttube/1
  Tinj/1 -> Mux1/4, Mux2/2
  ht/1 -> Mux1/5, Mux2/4
  Mux1/1 -> order/1, C*Cp/1
  Pair_in/1 -> Mux1/1
  Tair_in/1 -> Mux1/2, Mux2/1
  Uair_in/1 -> Mux1/3
  order/1 -> Mux2/5, in1/1
  Mux2/1 -> func/1
  Ttube/1 -> Mux2/3
  C*Cp/1 -> Divide/2
  Constant1/1 -> Manual Switch2/2
  Divide/1 -> Manual Switch2/1
  Manual Switch2/1 -> dot x19/1

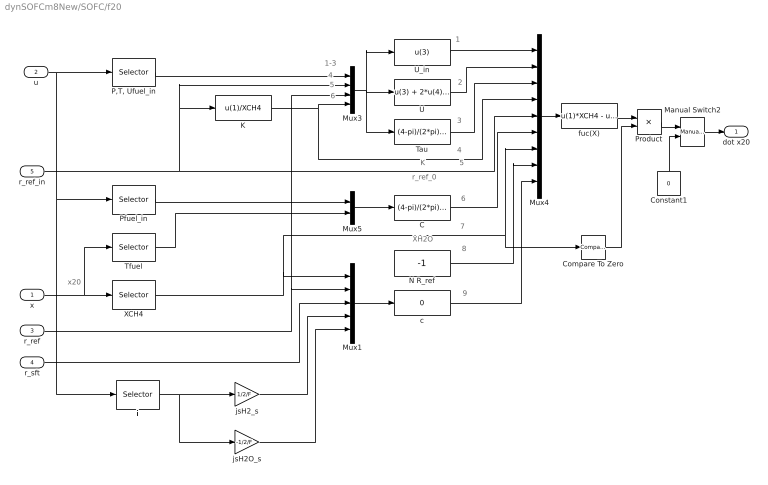
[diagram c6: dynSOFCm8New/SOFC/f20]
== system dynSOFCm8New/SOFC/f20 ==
  note: 1-3
  note: 4
  note: 5
  note: 6
  note: x20
  note: K
  note: XH2O
  note: 1
  note: 2
  note: 3
  note: 4
  note: 5
  note: 6
  note: 7
  note: 8
  note: r_ref_0
  note: 9
  x : Inport
  u : Inport  Port=2
  r_ref : Inport  Port=3
  r_sft : Inport  Port=4
  r_ref_in : Inport  Port=5
  C : Fcn  Expr=(4-pi)/(2*pi)*r3 * u(1) / ( R * u(2) )
  Compare To Zero : simulink/Logic and Bit Operations/Compare To Zero  relop=>=  LogicOutDataTypeMode=uint8  ZeroCross=off
  Constant1 : Constant  Orientation=up  Value=0
  K : Fcn  Expr=u(1)/XCH4
  Manual Switch2 : simulink/Signal Routing/Manual Switch  sw=1  action=0
  Mux1 : Mux  Inputs=5
  Mux3 : Mux
  Mux4 : Mux  Inputs=9
  Mux5 : Mux  Inputs=2
  N R_ref : Constant  Value=-1
  "P,T, Ufuel_in" : Selector  Elements=[2 3 4]  InputPortWidth=7
  Pfuel_in : Selector  Elements=[2]  InputPortWidth=7
  Product : Product
  Tau : Fcn  Expr=(4-pi)/(2*pi)*r3 * u(1) /R/u(2) * u(3) / u(6)
  Tfuel : Selector  Elements=[17]  InputPortWidth=25
  U : Fcn  Expr=u(3) + 2*u(4)*u(3)/u(6) * ( 1- exp( -X/((4-pi)/(2*pi)*r3 * u(1) /R/u(2) * u(3) / u(6)) ) )
  U_in : Fcn  Expr=u(3)
  XCH4 : Selector  Elements=[20]  InputPortWidth=25
  c : Fcn  Expr=0
  fuc(X) : Fcn  Expr=u(1)*XCH4 - u(2)*u(7) + u(8)/u(6)*u(3)*u(5)*( 1 - exp(-X/u(3)) ) + u(9)/u(6)*X
  i : Selector  Elements=[1]  InputPortWidth=7
  jsH2O_s : Gain  Gain=-1/2/F
  jsH2_s : Gain  Gain=1/2/F
  dot x20 : Outport
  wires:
  Tfuel/1 -> Mux5/2
  Pfuel_in/1 -> Mux5/1
  x/1 -> XCH4/1, Tfuel/1
  "P,T, Ufuel_in"/1 -> Mux3/1
  u/1 -> "P,T, Ufuel_in"/1, i/1, Pfuel_in/1
  Mux1/1 -> c/1
  r_ref_in/1 -> K/1, Mux3/2, Mux4/5
  Mux4/1 -> fuc(X)/1
  Mux5/1 -> C/1
  XCH4/1 -> Mux1/1, Mux4/7, Compare To Zero/1
  Constant1/1 -> Manual Switch2/2
  Manual Switch2/1 -> dot x20/1
  jsH2_s/1 -> Mux1/4
  jsH2O_s/1 -> Mux1/5
  r_ref/1 -> Mux3/3, Mux1/2
  r_sft/1 -> Mux1/3
  i/1 -> jsH2_s/1, jsH2O_s/1
  K/1 -> Mux3/4, Mux4/4
  C/1 -> Mux4/6
  N R_ref/1 -> Mux4/8
  c/1 -> Mux4/9
  Mux3/1 -> U/1, U_in/1, Tau/1
  U_in/1 -> Mux4/1
  U/1 -> Mux4/2
  Tau/1 -> Mux4/3
  fuc(X)/1 -> Product/1
  Compare To Zero/1 -> Product/2
  Product/1 -> Manual Switch2/1

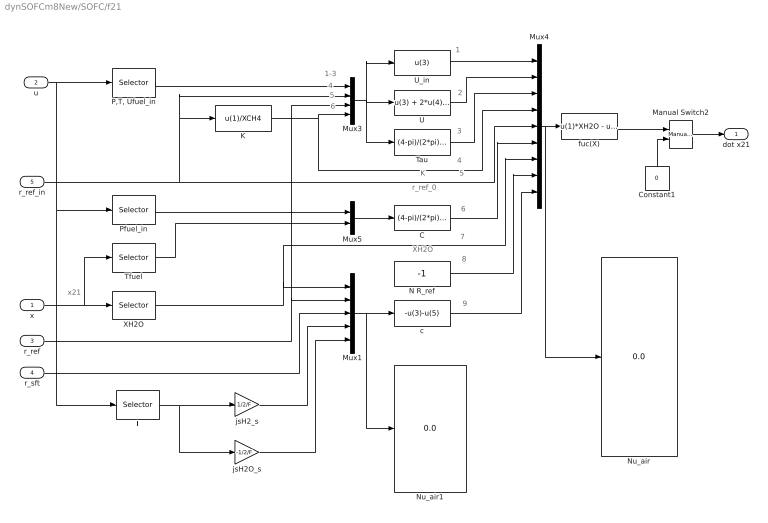
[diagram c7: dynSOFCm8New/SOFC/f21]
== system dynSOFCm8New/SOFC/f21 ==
  note: 1-3
  note: 4
  note: 5
  note: 6
  note: x21
  note: K
  note: XH2O
  note: 1
  note: 2
  note: 3
  note: 4
  note: 5
  note: 6
  note: 7
  note: 8
  note: r_ref_0
  note: 9
  x : Inport
  u : Inport  Port=2
  r_ref : Inport  Port=3
  r_sft : Inport  Port=4
  r_ref_in : Inport  Port=5
  C : Fcn  Expr=(4-pi)/(2*pi)*r3 * u(1) / ( R * u(2) )
  Constant1 : Constant  Orientation=up  Value=0
  K : Fcn  Expr=u(1)/XCH4
  Manual Switch2 : simulink/Signal Routing/Manual Switch  sw=1  action=0
  Mux1 : Mux  Inputs=5
  Mux3 : Mux
  Mux4 : Mux  Inputs=9
  Mux5 : Mux  Inputs=2
  N R_ref : Constant  Value=-1
  Nu_air : Display
  Nu_air1 : Display
  "P,T, Ufuel_in" : Selector  Elements=[2 3 4]  InputPortWidth=7
  Pfuel_in : Selector  Elements=[2]  InputPortWidth=7
  Tau : Fcn  Expr=(4-pi)/(2*pi)*r3 * u(1) /R/u(2) * u(3) / u(6)
  Tfuel : Selector  Elements=[17]  InputPortWidth=25
  U : Fcn  Expr=u(3) + 2*u(4)*u(3)/u(6) * ( 1- exp( -X/((4-pi)/(2*pi)*r3 * u(1) /R/u(2) * u(3) / u(6)) ) )
  U_in : Fcn  Expr=u(3)
  XH2O : Selector  Elements=[21]  InputPortWidth=25
  c : Fcn  Expr=-u(3)-u(5)
  fuc(X) : Fcn  Expr=u(1)*XH2O - u(2)*u(7) + u(8)/u(6)*u(3)*u(5)*( 1 - exp(-X/u(3)) ) + u(9)/u(6)*X
  i : Selector  Elements=[1]  InputPortWidth=7
  jsH2O_s : Gain  Gain=-1/2/F
  jsH2_s : Gain  Gain=1/2/F
  dot x21 : Outport
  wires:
  Constant1/1 -> Manual Switch2/2
  Manual Switch2/1 -> dot x21/1
  Tfuel/1 -> Mux5/2
  Pfuel_in/1 -> Mux5/1
  x/1 -> XH2O/1, Tfuel/1
  "P,T, Ufuel_in"/1 -> Mux3/1
  u/1 -> "P,T, Ufuel_in"/1, i/1, Pfuel_in/1
  Mux1/1 -> c/1, Nu_air1/1
  r_ref_in/1 -> K/1, Mux3/2, Mux4/5
  Mux4/1 -> fuc(X)/1, Nu_air/1
  Mux5/1 -> C/1
  fuc(X)/1 -> Manual Switch2/1
  XH2O/1 -> Mux1/1, Mux4/7
  jsH2_s/1 -> Mux1/4
  jsH2O_s/1 -> Mux1/5
  r_ref/1 -> Mux3/3, Mux1/2
  r_sft/1 -> Mux1/3
  i/1 -> jsH2_s/1, jsH2O_s/1
  K/1 -> Mux3/4, Mux4/4
  C/1 -> Mux4/6
  N R_ref/1 -> Mux4/8
  c/1 -> Mux4/9
  Mux3/1 -> U/1, U_in/1, Tau/1
  U_in/1 -> Mux4/1
  U/1 -> Mux4/2
  Tau/1 -> Mux4/3

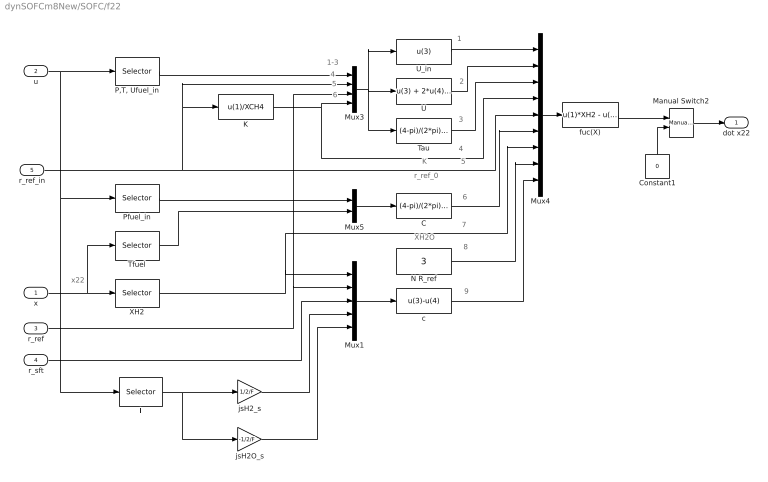
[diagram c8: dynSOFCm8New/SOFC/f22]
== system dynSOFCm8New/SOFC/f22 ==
  note: 1-3
  note: 4
  note: 5
  note: 6
  note: x22
  note: K
  note: XH2O
  note: 1
  note: 2
  note: 3
  note: 4
  note: 5
  note: 6
  note: 7
  note: 8
  note: r_ref_0
  note: 9
  x : Inport
  u : Inport  Port=2
  r_ref : Inport  Port=3
  r_sft : Inport  Port=4
  r_ref_in : Inport  Port=5
  C : Fcn  Expr=(4-pi)/(2*pi)*r3 * u(1) / ( R * u(2) )
  Constant1 : Constant  Orientation=up  Value=0
  K : Fcn  Expr=u(1)/XCH4
  Manual Switch2 : simulink/Signal Routing/Manual Switch  sw=1  action=0
  Mux1 : Mux  Inputs=5
  Mux3 : Mux
  Mux4 : Mux  Inputs=9
  Mux5 : Mux  Inputs=2
  N R_ref : Constant  Value=3
  "P,T, Ufuel_in" : Selector  Elements=[2 3 4]  InputPortWidth=7
  Pfuel_in : Selector  Elements=[2]  InputPortWidth=7
  Tau : Fcn  Expr=(4-pi)/(2*pi)*r3 * u(1) /R/u(2) * u(3) / u(6)
  Tfuel : Selector  Elements=[17]  InputPortWidth=25
  U : Fcn  Expr=u(3) + 2*u(4)*u(3)/u(6) * ( 1- exp( -X/((4-pi)/(2*pi)*r3 * u(1) /R/u(2) * u(3) / u(6)) ) )
  U_in : Fcn  Expr=u(3)
  XH2 : Selector  Elements=[22]  InputPortWidth=25
  c : Fcn  Expr=u(3)-u(4)
  fuc(X) : Fcn  Expr=u(1)*XH2 - u(2)*u(7) + u(8)/u(6)*u(3)*u(5)*( 1 - exp(-X/u(3)) ) + u(9)/u(6)*X
  i : Selector  Elements=[1]  InputPortWidth=7
  jsH2O_s : Gain  Gain=-1/2/F
  jsH2_s : Gain  Gain=1/2/F
  dot x22 : Outport
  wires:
  Constant1/1 -> Manual Switch2/2
  Manual Switch2/1 -> dot x22/1
  Tfuel/1 -> Mux5/2
  Pfuel_in/1 -> Mux5/1
  "P,T, Ufuel_in"/1 -> Mux3/1
  u/1 -> "P,T, Ufuel_in"/1, i/1, Pfuel_in/1
  Mux1/1 -> c/1
  r_ref_in/1 -> K/1, Mux3/2, Mux4/5
  Mux4/1 -> fuc(X)/1
  Mux5/1 -> C/1
  fuc(X)/1 -> Manual Switch2/1
  XH2/1 -> Mux1/1, Mux4/7
  jsH2_s/1 -> Mux1/4
  jsH2O_s/1 -> Mux1/5
  r_ref/1 -> Mux3/3, Mux1/2
  r_sft/1 -> Mux1/3
  i/1 -> jsH2_s/1, jsH2O_s/1
  K/1 -> Mux3/4, Mux4/4
  C/1 -> Mux4/6
  N R_ref/1 -> Mux4/8
  c/1 -> Mux4/9
  Mux3/1 -> U/1, U_in/1, Tau/1
  U_in/1 -> Mux4/1
  U/1 -> Mux4/2
  Tau/1 -> Mux4/3
  x/1 -> XH2/1, Tfuel/1

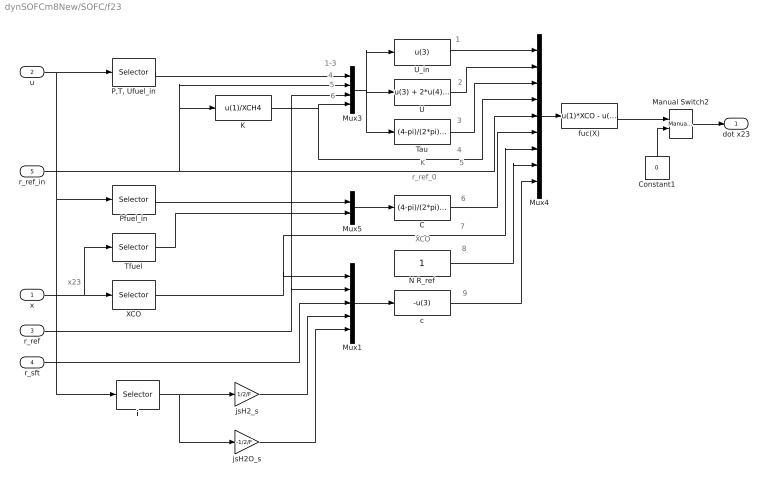
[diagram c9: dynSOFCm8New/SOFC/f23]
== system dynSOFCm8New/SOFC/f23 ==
  note: 1-3
  note: 4
  note: 5
  note: 6
  note: x23
  note: K
  note: XCO
  note: 1
  note: 2
  note: 3
  note: 4
  note: 5
  note: 6
  note: 7
  note: 8
  note: r_ref_0
  note: 9
  x : Inport
  u : Inport  Port=2
  r_ref : Inport  Port=3
  r_sft : Inport  Port=4
  r_ref_in : Inport  Port=5
  C : Fcn  Expr=(4-pi)/(2*pi)*r3 * u(1) / ( R * u(2) )
  Constant1 : Constant  Orientation=up  Value=0
  K : Fcn  Expr=u(1)/XCH4
  Manual Switch2 : simulink/Signal Routing/Manual Switch  sw=1  action=0
  Mux1 : Mux  Inputs=5
  Mux3 : Mux
  Mux4 : Mux  Inputs=9
  Mux5 : Mux  Inputs=2
  N R_ref : Constant
  "P,T, Ufuel_in" : Selector  Elements=[2 3 4]  InputPortWidth=7
  Pfuel_in : Selector  Elements=[2]  InputPortWidth=7
  Tau : Fcn  Expr=(4-pi)/(2*pi)*r3 * u(1) /R/u(2) * u(3) / u(6)
  Tfuel : Selector  Elements=[17]  InputPortWidth=25
  U : Fcn  Expr=u(3) + 2*u(4)*u(3)/u(6) * ( 1- exp( -X/((4-pi)/(2*pi)*r3 * u(1) /R/u(2) * u(3) / u(6)) ) )
  U_in : Fcn  Expr=u(3)
  XCO : Selector  Elements=[23]  InputPortWidth=25
  c : Fcn  Expr=-u(3)
  fuc(X) : Fcn  Expr=u(1)*XCO - u(2)*u(7) + u(8)/u(6)*u(3)*u(5)*( 1 - exp(-X/u(3)) ) + u(9)/u(6)*X
  i : Selector  Elements=[1]  InputPortWidth=7
  jsH2O_s : Gain  Gain=-1/2/F
  jsH2_s : Gain  Gain=1/2/F
  dot x23 : Outport
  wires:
  Constant1/1 -> Manual Switch2/2
  Manual Switch2/1 -> dot x23/1
  Tfuel/1 -> Mux5/2
  Pfuel_in/1 -> Mux5/1
  x/1 -> XCO/1, Tfuel/1
  "P,T, Ufuel_in"/1 -> Mux3/1
  u/1 -> "P,T, Ufuel_in"/1, i/1, Pfuel_in/1
  Mux1/1 -> c/1
  r_ref_in/1 -> K/1, Mux3/2, Mux4/5
  Mux4/1 -> fuc(X)/1
  Mux5/1 -> C/1
  fuc(X)/1 -> Manual Switch2/1
  XCO/1 -> Mux1/1, Mux4/7
  jsH2_s/1 -> Mux1/4
  jsH2O_s/1 -> Mux1/5
  r_ref/1 -> Mux3/3, Mux1/2
  r_sft/1 -> Mux1/3
  i/1 -> jsH2_s/1, jsH2O_s/1
  K/1 -> Mux3/4, Mux4/4
  C/1 -> Mux4/6
  N R_ref/1 -> Mux4/8
  c/1 -> Mux4/9
  Mux3/1 -> U/1, U_in/1, Tau/1
  U_in/1 -> Mux4/1
  U/1 -> Mux4/2
  Tau/1 -> Mux4/3

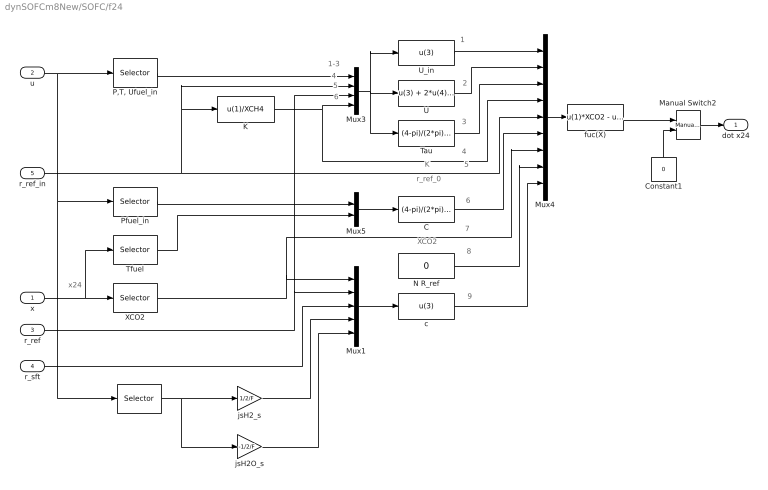
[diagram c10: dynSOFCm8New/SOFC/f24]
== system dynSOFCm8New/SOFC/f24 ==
  note: 1-3
  note: 4
  note: 5
  note: 6
  note: x24
  note: K
  note: XCO2
  note: 1
  note: 2
  note: 3
  note: 4
  note: 5
  note: 6
  note: 7
  note: 8
  note: r_ref_0
  note: 9
  x : Inport
  u : Inport  Port=2
  r_ref : Inport  Port=3
  r_sft : Inport  Port=4
  r_ref_in : Inport  Port=5
  C : Fcn  Expr=(4-pi)/(2*pi)*r3 * u(1) / ( R * u(2) )
  Constant1 : Constant  Orientation=up  Value=0
  K : Fcn  Expr=u(1)/XCH4
  Manual Switch2 : simulink/Signal Routing/Manual Switch  sw=1  action=0
  Mux1 : Mux  Inputs=5
  Mux3 : Mux
  Mux4 : Mux  Inputs=9
  Mux5 : Mux  Inputs=2
  N R_ref : Constant  Value=0
  "P,T, Ufuel_in" : Selector  Elements=[2 3 4]  InputPortWidth=7
  Pfuel_in : Selector  Elements=[2]  InputPortWidth=7
  Tau : Fcn  Expr=(4-pi)/(2*pi)*r3 * u(1) /R/u(2) * u(3) / u(6)
  Tfuel : Selector  Elements=[17]  InputPortWidth=25
  U : Fcn  Expr=u(3) + 2*u(4)*u(3)/u(6) * ( 1- exp( -X/((4-pi)/(2*pi)*r3 * u(1) /R/u(2) * u(3) / u(6)) ) )
  U_in : Fcn  Expr=u(3)
  XCO2 : Selector  Elements=[24]  InputPortWidth=25
  c : Fcn  Expr=u(3)
  fuc(X) : Fcn  Expr=u(1)*XCO2 - u(2)*u(7) + u(8)/u(6)*u(3)*u(5)*( 1 - exp(-X/u(3)) ) + u(9)/u(6)*X
  i : Selector  Elements=[1]  InputPortWidth=7
  jsH2O_s : Gain  Gain=-1/2/F
  jsH2_s : Gain  Gain=1/2/F
  dot x24 : Outport
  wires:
  Constant1/1 -> Manual Switch2/2
  Manual Switch2/1 -> dot x24/1
  Tfuel/1 -> Mux5/2
  Pfuel_in/1 -> Mux5/1
  "P,T, Ufuel_in"/1 -> Mux3/1
  u/1 -> "P,T, Ufuel_in"/1, i/1, Pfuel_in/1
  Mux1/1 -> c/1
  r_ref_in/1 -> K/1, Mux3/2, Mux4/5
  Mux4/1 -> fuc(X)/1
  Mux5/1 -> C/1
  fuc(X)/1 -> Manual Switch2/1
  XCO2/1 -> Mux1/1, Mux4/7
  jsH2_s/1 -> Mux1/4
  jsH2O_s/1 -> Mux1/5
  r_ref/1 -> Mux3/3, Mux1/2
  r_sft/1 -> Mux1/3
  i/1 -> jsH2_s/1, jsH2O_s/1
  K/1 -> Mux3/4, Mux4/4
  C/1 -> Mux4/6
  N R_ref/1 -> Mux4/8
  c/1 -> Mux4/9
  Mux3/1 -> U/1, U_in/1, Tau/1
  U_in/1 -> Mux4/1
  U/1 -> Mux4/2
  Tau/1 -> Mux4/3
  x/1 -> XCO2/1, Tfuel/1

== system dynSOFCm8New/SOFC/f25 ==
  note: x4
  note: x18
  note: 1
  note: 4
  note: 5
  note: 2
  note: x25
  note: 3
  x : Inport
  u : Inport  Port=2
  C : Fcn  Expr=(r2^2-r1^2)/(2*r2) * u(1) / ( R * u(2) )
  Constant1 : Constant  Orientation=up  Value=0
  Divide : Product  Inputs=*/
  Manual Switch2 : simulink/Signal Routing/Manual Switch  sw=0  action=0
  Mux3 : Mux  Inputs=5
  Mux4 : Mux
  Mux5 : Mux  Inputs=2
  Pair_in : Selector  Elements=[5]  InputPortWidth=7
  Tair : Selector  Elements=[18]  InputPortWidth=25
  Tair_in : Selector  Elements=[6]  InputPortWidth=7
  Tb : Gain  Gain=1.01
  U/U_in : Fcn  Expr="1 - 1/2/(r2^2-r1^2)*(2*r1)  * R/u(1)/u(3) * u(4) * ( u(2) + u(5)  ) * X"
  Uair_in : Selector  Elements=[7]  InputPortWidth=7
  Ub : Gain  Gain=r0/(r2-r1)
  XO2 : Selector  Elements=[25]  InputPortWidth=25
  fuc(X) : Fcn  Expr=- u(3) + 1 - 0.79 * ( u(1) ^ u(2))
  jsO2 : Selector  Elements=[4]  InputPortWidth=25
  order : Fcn  Expr="- 2 * u(5)  / ( u(2)  + u(5)  )"
  dot x25 : Outport
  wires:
  Tair/1 -> Mux5/2, Mux3/5
  jsO2/1 -> Mux3/4, Mux4/4
  x/1 -> XO2/1, jsO2/1, Tair/1
  Mux3/1 -> U/U_in/1, order/1
  Mux4/1 -> fuc(X)/1
  U/U_in/1 -> Mux4/1
  Mux5/1 -> C/1
  fuc(X)/1 -> Divide/1
  C/1 -> Divide/2
  XO2/1 -> Mux4/3
  order/1 -> Mux4/2
  Uair_in/1 -> Ub/1
  Tair_in/1 -> Tb/1
  Pair_in/1 -> Mux3/1, Mux5/1
  Tb/1 -> Mux3/2
  Ub/1 -> Mux3/3
  u/1 -> Pair_in/1, Tair_in/1, Uair_in/1
  Divide/1 -> Manual Switch2/1
  Constant1/1 -> Manual Switch2/2
  Manual Switch2/1 -> dot x25/1

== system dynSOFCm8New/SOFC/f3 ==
  note: 1-2
  note: 3
  note: 4
  note: 5-8
  note: x2,3
  note: u1
  note: x22
  note: u2,3
  note: dot CbH2
  note: dot jsH2
  note: jsH2
  note: i
  x : Inport
  u : Inport  Port=2
  DH2 : Inport  Port=3
  CbH2 : Fcn  Expr=XH2 *u(2)/R/u(3)
  Derivative1 : Derivative
  Ex3 : Fcn  Expr=-u(5)*u(1) - u(6)*u(2) + u(5)/(2*F)*u(4) + u(7)*u(3)
  JsH2 : Selector  Elements=[2 3]  InputPortWidth=25
  Mux : Mux
  Mux1 : Mux
  Mux4 : Mux  Inputs=2
  Pfuel_in : Selector  Elements=[2 3]  InputPortWidth=7
  Transfer Fcn : TransferFcn  Denominator=[0.001 1]
  XH2 : Selector  Elements=[22 ]  InputPortWidth=25
  a1 : Fcn  Expr=24*u(1)^2/(La^4)
  a2 : Fcn  Expr=12*u(1)/(La^2)
  a3 : Fcn  Expr=24*u(1)^2/(La^3)
  a4 : Fcn  Expr=24*u(1)/(La^3)
  i : Selector  Elements=[1]  InputPortWidth=7
  dot x3 : Outport
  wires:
  x/1 -> JsH2/1, XH2/1
  DH2/1 -> a1/1, a2/1, a4/1, a3/1
  a1/1 -> Mux/1
  a2/1 -> Mux/2
  a3/1 -> Mux/3
  a4/1 -> Mux/4
  Mux1/1 -> Ex3/1
  Ex3/1 -> dot x3/1
  CbH2/1 -> Derivative1/1
  u/1 -> Pfuel_in/1, i/1
  JsH2/1 -> Mux1/1
  Derivative1/1 -> Transfer Fcn/1
  XH2/1 -> Mux4/1
  Pfuel_in/1 -> Mux4/2
  Mux4/1 -> CbH2/1
  i/1 -> Mux1/3
  Transfer Fcn/1 -> Mux1/2
  Mux/1 -> Mux1/4

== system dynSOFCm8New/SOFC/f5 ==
  note: 1-2
  note: 3
  note: 4
  note: 5-8
  note: x4,5
  note: u1
  note: 25
  note: u5,6
  note: dot CbO2
  note: dot jsO2
  note: jsO2
  note: i
  x : Inport
  u : Inport  Port=2
  DO2 : Inport  Port=3
  CbO2 : Fcn  Expr=XO2*u(2)/R/u(3)
  Derivative2 : Derivative
  Ex5 : Fcn  Expr=-u(5)*u(1) - u(6)*u(2) + u(5)/(4*F)*u(4) + u(7)*u(3)
  JsO2 : Selector  Elements=[4 5]  InputPortWidth=25
  Mux : Mux
  Mux4 : Mux
  Mux5 : Mux  Inputs=2
  Pair_in : Selector  Elements=[5 6]  InputPortWidth=7
  Transfer Fcn1 : TransferFcn  Denominator=[0.001 1]
  XO2 : Selector  Elements=[25 ]  InputPortWidth=25
  a1 : Fcn  Expr=24*u(1)^2/(Lc^4)
  a2 : Fcn  Expr=12*u(1)/(Lc^2)
  a3 : Fcn  Expr=24*u(1)^2/(Lc^3)
  a4 : Fcn  Expr=24*u(1)/(Lc^3)
  i : Selector  Elements=[1]  InputPortWidth=7
  dot x5 : Outport
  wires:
  a4/1 -> Mux/4
  a3/1 -> Mux/3
  a2/1 -> Mux/2
  a1/1 -> Mux/1
  DO2/1 -> a3/1, a4/1, a2/1, a1/1
  x/1 -> JsO2/1, XO2/1
  Mux4/1 -> Ex5/1
  Ex5/1 -> dot x5/1
  CbO2/1 -> Derivative2/1
  u/1 -> Pair_in/1, i/1
  JsO2/1 -> Mux4/1
  Derivative2/1 -> Transfer Fcn1/1
  XO2/1 -> Mux5/1
  Pair_in/1 -> Mux5/2
  Mux5/1 -> CbO2/1
  i/1 -> Mux4/3
  Transfer Fcn1/1 -> Mux4/2
  Mux/1 -> Mux4/4

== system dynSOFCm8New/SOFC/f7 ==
  note: 1-2
  note: 3
  note: 4
  note: 5-8
  note: x6,7
  note: u1
  note: x21
  note: u2,3
  note: dot CbH2O
  note: dot jsH2O
  note: jsH2O
  note: i
  x : Inport
  u : Inport  Port=2
  DH2O : Inport  Port=3
  CbH2O : Fcn  Expr=XH2O*u(2)/R/u(3)
  Derivative2 : Derivative
  Ex7 : Fcn  Expr=-u(5)*u(1) - u(6)*u(2) + u(5)/(2*F)*(-u(4)) + u(7)*u(3)
  JsH2O : Selector  Elements=[6 7]  InputPortWidth=25
  Mux : Mux
  Mux4 : Mux
  Mux5 : Mux  Inputs=2
  Pfuel_in : Selector  Elements=[2 3]  InputPortWidth=7
  Transfer Fcn1 : TransferFcn  Denominator=[0.001 1]
  XH2O : Selector  Elements=[ 21 ]  InputPortWidth=25
  a1 : Fcn  Expr=24*u(1)^2/(Lc^4)
  a2 : Fcn  Expr=12*u(1)/(Lc^2)
  a3 : Fcn  Expr=24*u(1)^2/(Lc^3)
  a4 : Fcn  Expr=24*u(1)/(Lc^3)
  i : Selector  Elements=[1]  InputPortWidth=7
  dot x7 : Outport
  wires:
  DH2O/1 -> a1/1, a2/1, a4/1, a3/1
  a1/1 -> Mux/1
  a2/1 -> Mux/2
  a3/1 -> Mux/3
  a4/1 -> Mux/4
  x/1 -> JsH2O/1, XH2O/1
  Mux4/1 -> Ex7/1
  Ex7/1 -> dot x7/1
  CbH2O/1 -> Derivative2/1
  u/1 -> Pfuel_in/1, i/1
  JsH2O/1 -> Mux4/1
  Derivative2/1 -> Transfer Fcn1/1
  XH2O/1 -> Mux5/1
  Pfuel_in/1 -> Mux5/2
  Mux5/1 -> CbH2O/1
  i/1 -> Mux4/3
  Transfer Fcn1/1 -> Mux4/2
  Mux/1 -> Mux4/4

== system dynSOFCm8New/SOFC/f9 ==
  note: 1-4
  note: 5
  note: 6
  note: 7-10
  note: x8,9,14,15
  note: u1
  note: x22
  note: u2
  note: pbH2
  note: dot ptH2
  note: ptH2
  note: i
  note: Vi
  note: Tcell
  x : Inport
  u : Inport  Port=2
  DH2 : Inport  Port=3
  Ex9 : Fcn  Expr="-u(7)*u(1) - u(8)*u(2)  + u(7)*u(5) - R*u(4)/(2*F)*( u(10)*u(6) + 4/La*(K*u(6)-u(3)) )"
  Mux : Mux
  Mux3 : Mux
  Mux4 : Mux  Inputs=2
  Pfuel_in : Selector  Elements=[2]  InputPortWidth=7
  XH2 : Selector  Elements=[22 ]  InputPortWidth=25
  a1 : Fcn  Expr=24*u(1)^2/(La^4)
  a2 : Fcn  Expr=12*u(1)/(La^2)
  a3 : Fcn  Expr=24*u(1)^2/(La^3)
  a4 : Fcn  Expr=24*u(1)/(La^3)
  i : Selector  Elements=[1]  InputPortWidth=7
  pbH2 : Fcn  Expr=u(2)*u(1)
  ptH2 : Selector  Elements=[8 9 14 15]  InputPortWidth=25
  dot x9 : Outport
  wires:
  a4/1 -> Mux/4
  a3/1 -> Mux/3
  a2/1 -> Mux/2
  a1/1 -> Mux/1
  DH2/1 -> a3/1, a4/1, a2/1, a1/1
  x/1 -> ptH2/1, XH2/1
  Mux3/1 -> Ex9/1
  Ex9/1 -> dot x9/1
  pbH2/1 -> Mux3/2
  u/1 -> Pfuel_in/1, i/1
  ptH2/1 -> Mux3/1
  XH2/1 -> Mux4/1
  Pfuel_in/1 -> Mux4/2
  Mux4/1 -> pbH2/1
  i/1 -> Mux3/3
  Mux/1 -> Mux3/4
